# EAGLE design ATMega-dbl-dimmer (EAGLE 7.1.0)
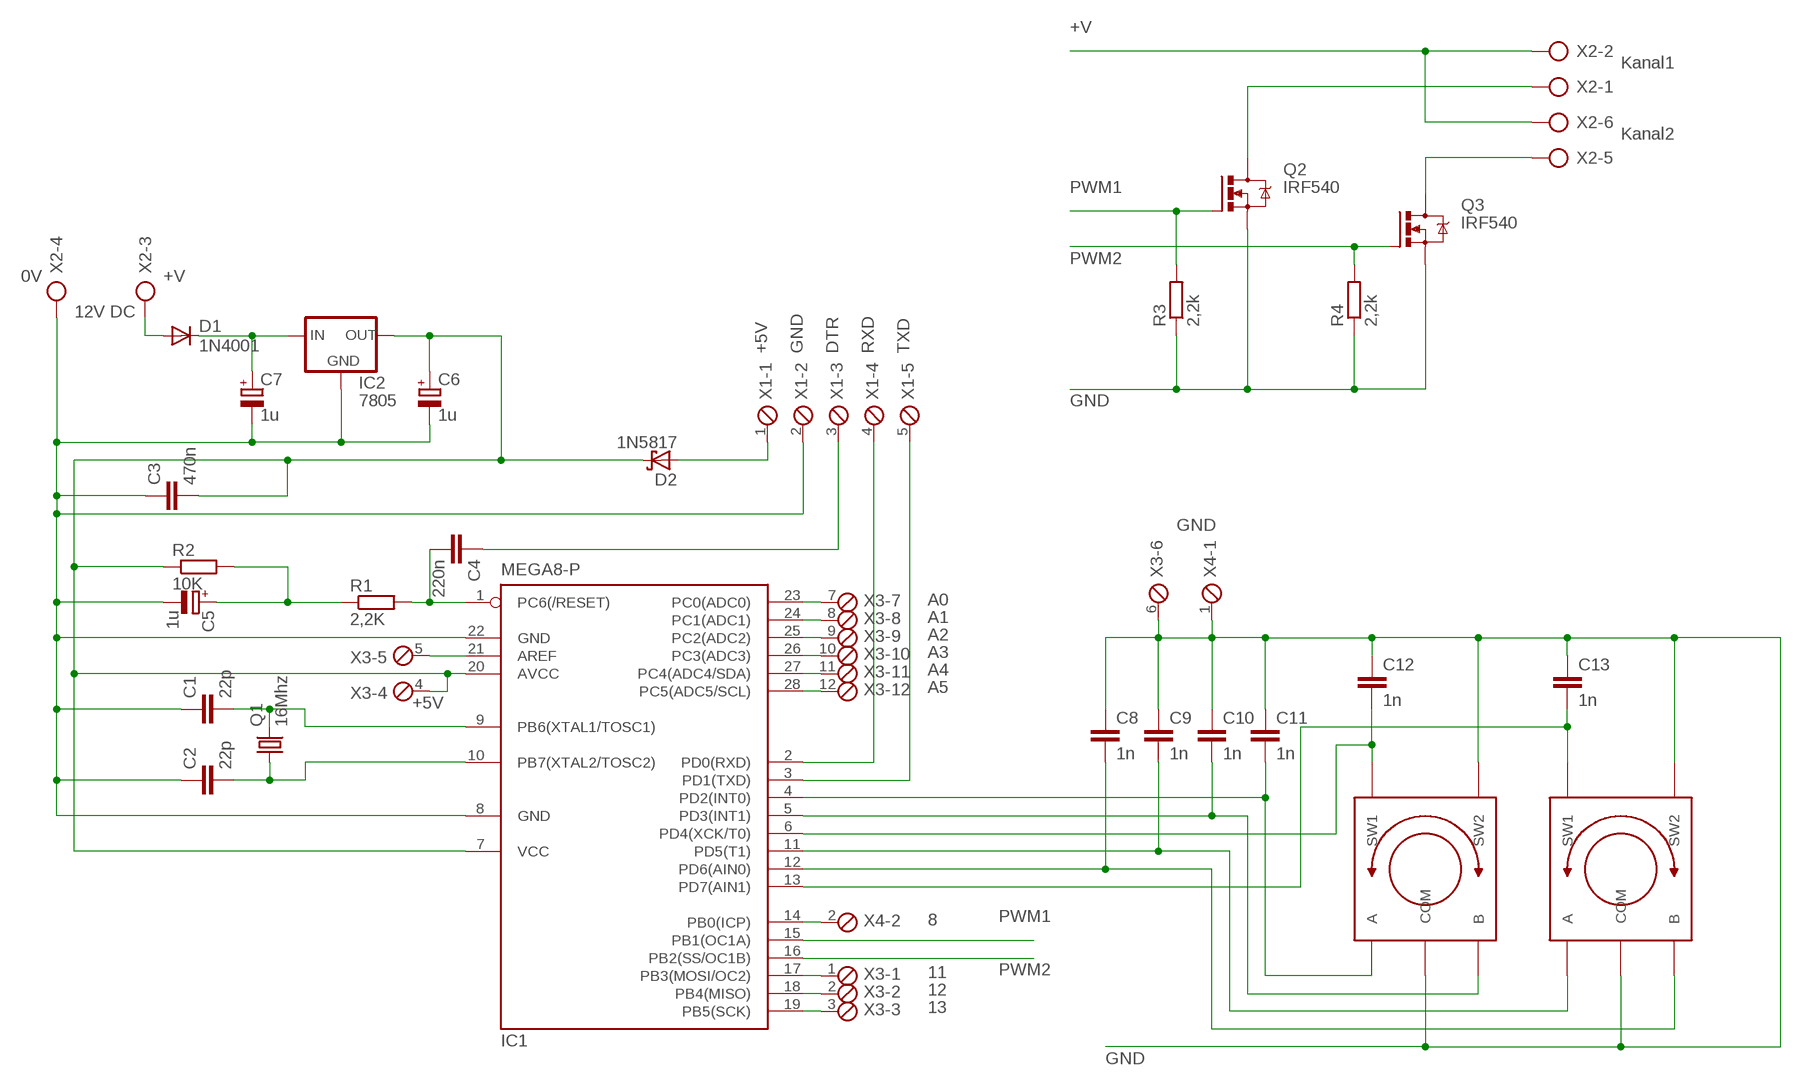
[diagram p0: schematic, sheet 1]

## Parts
C1  22p  C-EU025-025X050  [C025-025X050]
C2  22p  C-EU025-025X050  [C025-025X050]
C3  470n  C-EU075-042X103  [C075-042X103]
C4  220n  C-EU075-032X103  [C075-032X103]
C5  1u  CPOL-EUE5-6  [E5-6]
C6  1u  CPOL-EUE5-6  [E5-6]
C7  1u  CPOL-EUE5-6  [E5-6]
C8  1n  C-EU025-025X050  [C025-025X050]
C9  1n  C-EU025-025X050  [C025-025X050]
C10  1n  C-EU025-025X050  [C025-025X050]
C11  1n  C-EU025-025X050  [C025-025X050]
C12  1n  C-EU025-025X050  [C025-025X050]
C13  1n  C-EU025-025X050  [C025-025X050]
D1  1N4001  1N4004  [DO41-10]
D2  1N5817  1N5817-B  [DO41-7.6]
IC1  MEGA8-P  [DIL28-3]
IC2  7805  78XXS  [78XXS]
Q1  16Mhz  CRYSTALHC49S  [HC49/S]
Q2  IRF540  [TO220BV]
Q3  IRF540  [TO220BV]
R1  2,2K  R-EU_0207/7  [0207/7]
R2  10K  R-EU_0207/7  [0207/7]
R3  2,2k  R-EU_0207/7  [0207/7]
R4  2,2k  R-EU_0207/7  [0207/7]
S1  ROTARY-ENCODER  [RT-ENC-H]
S2  ROTARY-ENCODER  [RT-ENC-H]
X1  MPT5  [5POL254]
X2  AK300/6  [AK300/6]
X3  MPT12  [12POL254]
X4  MPT2  [2POL254]

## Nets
+5V: C3.2 C6.+ D2.C IC1.7(VCC) IC1.20(AVCC) IC2.OUT R2.1 X3.4
+V: D1.A X2.2 X2.3 X2.6
+V1: C7.+ D1.C IC2.IN
GND: C1.1 C2.1 C3.1 C5.- C6.- C7.- C8.1 C9.1 C10.1 C11.1 C12.1 C13.1 IC1.8(GND) IC1.22(GND) IC2.GND Q2.S Q3.S R3.1 R4.1 S1.P$2(COM) S1.P$5(SW2) S2.P$2(COM) S2.P$5(SW2) X1.2 X2.4 X3.6 X4.1
N$1: C1.2 IC1.9(PB6(XTAL1/TOSC1)) Q1.2
N$2: C2.2 IC1.10(PB7(XTAL2/TOSC2)) Q1.1
N$3: C4.2 IC1.1(PC6(/RESET)) R1.2
N$4: C5.+ R1.1 R2.2
N$7: IC1.2(PD0(RXD)) X1.4
N$8: IC1.3(PD1(TXD)) X1.5
N$9: C4.1 X1.3
N$10: C12.2 IC1.6(PD4(XCK/T0)) S1.P$4(SW1)
N$11: C13.2 IC1.13(PD7(AIN1)) S2.P$4(SW1)
N$12: C11.2 IC1.4(PD2(INT0)) S1.P$1(A)
N$13: C10.2 IC1.5(PD3(INT1)) S1.P$3(B)
N$14: C9.2 IC1.11(PD5(T1)) S2.P$1(A)
N$15: C8.2 IC1.12(PD6(AIN0)) S2.P$3(B)
N$16: Q3.D X2.5
N$17: Q2.D X2.1
N$19: IC1.21(AREF) X3.5
N$20: IC1.23(PC0(ADC0)) X3.7
N$21: IC1.24(PC1(ADC1)) X3.8
N$22: IC1.25(PC2(ADC2)) X3.9
N$23: IC1.26(PC3(ADC3)) X3.10
N$24: IC1.27(PC4(ADC4/SDA)) X3.11
N$25: IC1.28(PC5(ADC5/SCL)) X3.12
N$26: IC1.17(PB3(MOSI/OC2)) X3.1
N$27: IC1.18(PB4(MISO)) X3.2
N$28: IC1.19(PB5(SCK)) X3.3
N$29: IC1.14(PB0(ICP)) X4.2
N$30: D2.A X1.1
PWM1: IC1.15(PB1(OC1A)) Q2.G R3.2
PWM2: IC1.16(PB2(SS/OC1B)) Q3.G R4.2

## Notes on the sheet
- +V
- Kanal1
- Kanal2
- PWM1
- PWM2
- 0V | +V
- 12V DC
- +5V | GND | DTR | RXD | TXD
- GND
- GND
- A0
  A1
  A2
  A3
  A4
  A5
- +5V
- PWM1
- PWM2
- 8
  
  
  11
  12
  13
- GND

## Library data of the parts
C1-C4 C8-C13 = rcl:C-EU: CAPACITOR, European symbol
C5-C7 = rcl:CPOL-EU: POLARIZED CAPACITOR, European symbol
D1 = diode:1N4004: DIODE
D2 = diode:1N581*: 1.0A SCHOTTKY BARRIER RECTIFIER
IC1 = atmel:MEGA8-P: MICROCONTROLLER 8 Kbytes FLASH, 1 kbytes SRAM, 512 bytes EEPROM, USART, 4-channel 10 bit ADC, 2-channel 8 bit ADC Pin compatible with Atmega48, ATMega88, ATMega168 Source: avr.lbr; OC_FARNELL: unknown; OC_NEWARK: unknown
IC2 = v-reg:78XXS: VOLTAGE REGULATOR
Q1 = crystal:CRYSTAL: CRYSTAL; OC_FARNELL: 1667008; OC_NEWARK: unknown
Q2 Q3 = transistor-power:IRF540: HEXFET Power MOSFET
R1-R4 = rcl:R-EU_: RESISTOR, European symbol
S1 S2 = tormod:ROTARY-ENCODER
X1 = con-phoenix-254:MPT5: PHOENIX CONNECTOR; OC_FARNELL: unknown; OC_NEWARK: unknown
X2 = con-ptr500:AK300/6: CONNECTOR; OC_FARNELL: unknown; OC_NEWARK: unknown
X3 = con-phoenix-254:MPT12: PHOENIX CONNECTOR; OC_FARNELL: unknown; OC_NEWARK: unknown
X4 = con-phoenix-254:MPT2: PHOENIX CONNECTOR; OC_FARNELL: unknown; OC_NEWARK: unknown

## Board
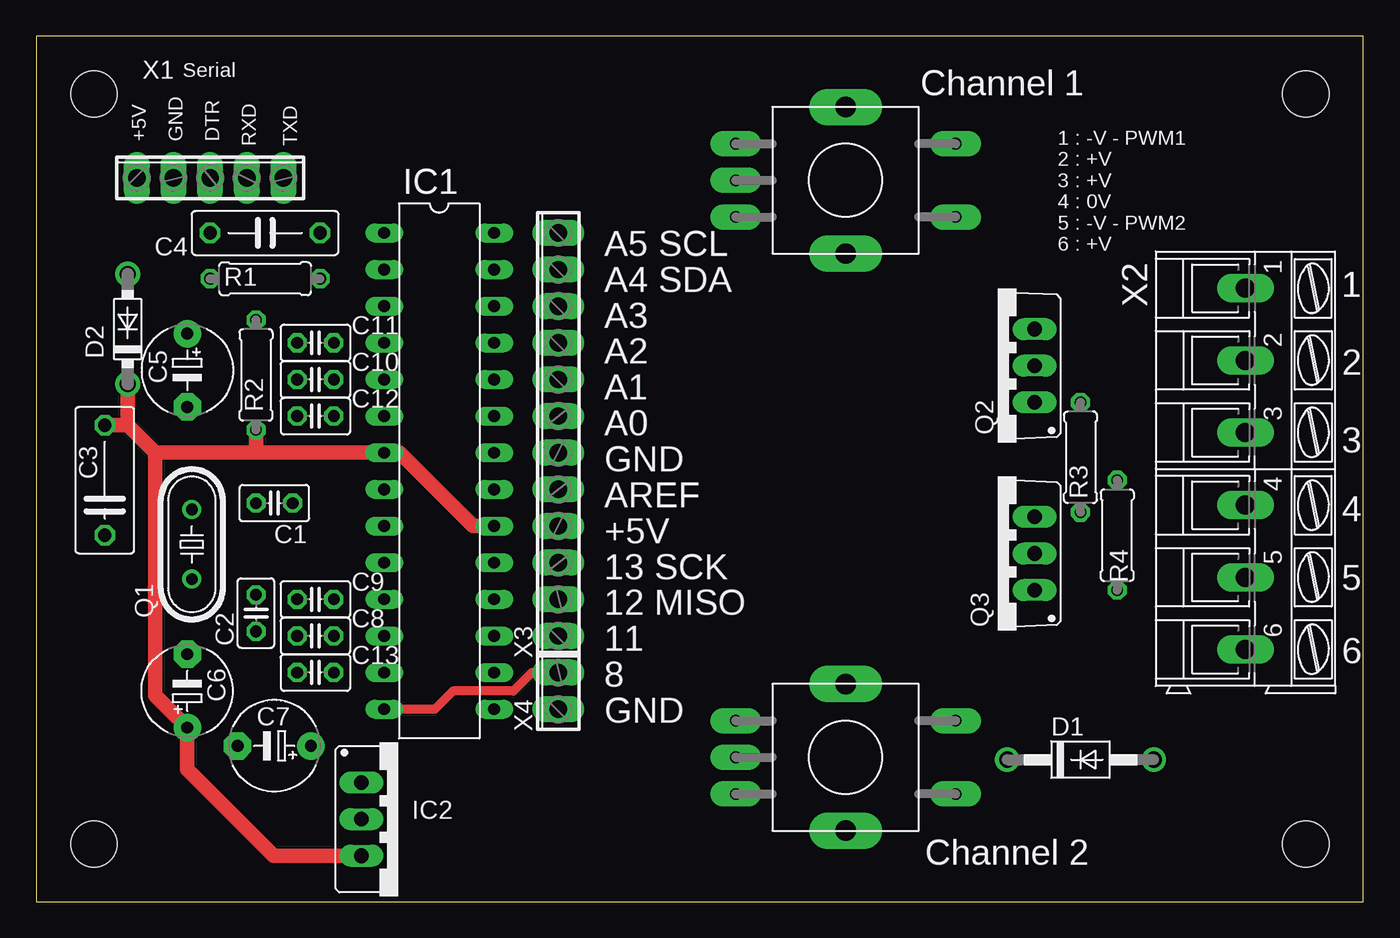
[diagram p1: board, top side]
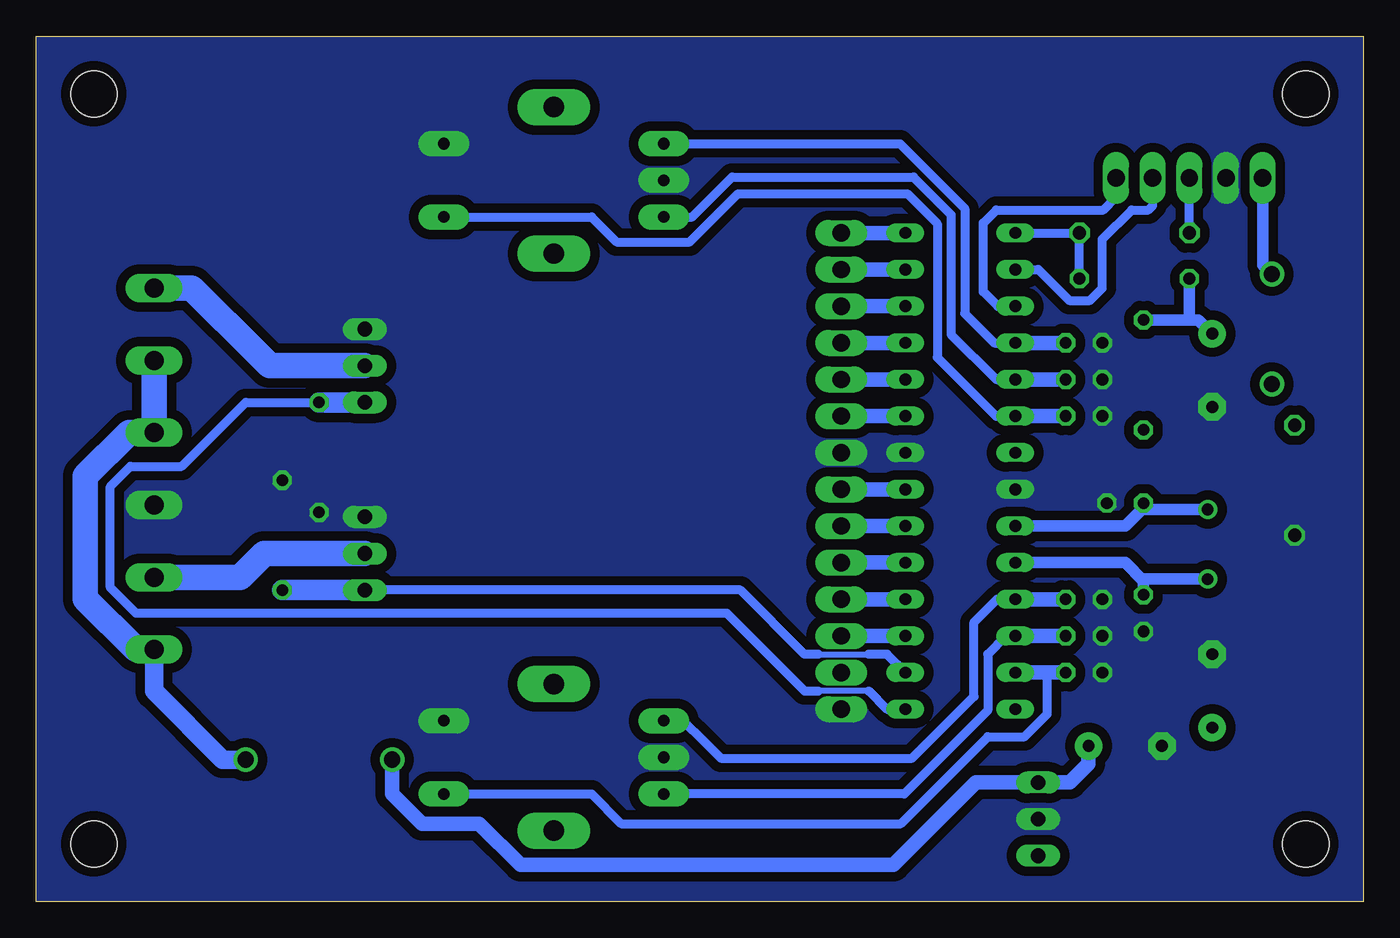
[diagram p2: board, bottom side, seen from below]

Size 92 x 60 mm. Coordinates in mm from the lower left corner, seen from the top.
Outline: 0,0 92,0 92,60 0,60 0,0
Copper layers (1*16): Top 0.035mm / dielectric 1.5mm / Bottom 0.035mm
Design rules "default *": minimum track width 10mil, minimum drill 24mil, track to track 8mil, track to pad 8mil, pad to pad 8mil, via to via 8mil, smd to smd 8mil, copper to edge 0mil, drill to drill 8mil, minimum pad ring 10mil, minimum via ring 8mil, stop-mask expansion 4mil, vias tented up to drill 0mil, thermal gap 10mil
Holes 3.2 mm at 4,56 88,56 88,4 4,4

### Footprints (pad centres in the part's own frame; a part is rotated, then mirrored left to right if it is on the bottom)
C025-025X050 = drill 0.813 octagon: 1 -1.27,0; 2 1.27,0
C075-042X103 = drill 0.914 octagon: 1 -3.81,0; 2 3.81,0
C075-032X103 = drill 0.914 octagon: 1 -3.81,0; 2 3.81,0
E5-6 = drill 0.813 pad 1.905: + -2.54,0 | drill 0.813 pad 1.905 octagon: - 2.54,0
DO41-10 = drill 1.118: A 5.08,0; C -5.08,0
DO41-7.6 = drill 1.1 pad 1.7: A 3.81,0; C -3.81,0
DIL28-3 = drill 0.813 long: 1 -16.51,-3.81; 2 -13.97,-3.81; 3 -11.43,-3.81; 4 -8.89,-3.81; 5 -6.35,-3.81; 6 -3.81,-3.81; 7 -1.27,-3.81; 8 1.27,-3.81; 9 3.81,-3.81; 10 6.35,-3.81; 11 8.89,-3.81; 12 11.43,-3.81; 13 13.97,-3.81; 14 16.51,-3.81; 15 16.51,3.81; 16 13.97,3.81; 17 11.43,3.81; 18 8.89,3.81; 19 6.35,3.81; 20 3.81,3.81; 21 1.27,3.81; 22 -1.27,3.81; 23 -3.81,3.81; 24 -6.35,3.81; 25 -8.89,3.81; 26 -11.43,3.81; 27 -13.97,3.81; 28 -16.51,3.81
78XXS = drill 1.016 long: GND 0,-2.54; IN -2.54,-2.54; OUT 2.54,-2.54
HC49/S = drill 0.813: 1 -2.413,0; 2 2.413,0
TO220BV = drill 1.016 long: D 0,-2.54; G -2.54,-2.54; S 2.54,-2.54
0207/7 = drill 0.813 octagon: 1 -3.81,0; 2 3.81,0
RT-ENC-H = drill 0.8 pad 1.778 long: P$1 -7.62,2.54; P$2 -7.62,0; P$3 -7.62,-2.54; P$4 7.62,-2.54; P$5 7.62,2.54 | drill 1.4 pad 2.54 long: P$6 0,5.08; P$7 0,-5.08
5POL254 = drill 1.2 long: 1 -5.08,0; 2 -2.54,0; 3 0,0; 4 2.54,0; 5 5.08,0
AK300/6 = drill 1.321 long: 1 -12.522,0; 2 -7.518,0; 3 -2.515,0; 4 2.515,0; 5 7.518,0; 6 12.522,0
12POL254 = drill 1.2 long: 1 -13.97,0; 2 -11.43,0; 3 -8.89,0; 4 -6.35,0; 5 -3.81,0; 6 -1.27,0; 7 1.27,0; 8 3.81,0; 9 6.35,0; 10 8.89,0; 11 11.43,0; 12 13.97,0
2POL254 = drill 1.2 long: 1 -1.27,0; 2 1.27,0

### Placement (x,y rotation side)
C1  16.51,27.62 180 top
C2  15.24,20 90 top
C3  4.76,29.21 90 top
C4  15.88,46.35 0 top
C5  10.48,36.83 270 top
C6  10.48,14.61 90 top
C7  16.51,10.79 180 top
C8  19.37,18.41 0 top
C9  19.37,20.95 0 top
C10  19.37,36.2 0 top
C11  19.37,38.73 0 top
C12  19.37,33.66 0 top
C13  19.37,15.88 0 top
D1  72.39,9.84 0 top
D2  6.35,39.69 90 top
IC1  27.94,29.84 270 top
IC2  25.08,5.71 270 top
Q1  10.79,24.77 90 top
Q2  66.67,37.15 90 top
Q3  66.67,24.13 90 top
R1  15.88,43.18 0 top
R2  15.24,36.51 90 top
R3  72.39,30.8 90 top
R4  74.93,25.4 270 top
S1  56.11,50 0 top
S2  56.11,10 0 top
X1  12.06,50.16 0 top
X2  83.82,30 270 top
X3  36.2,32.38 90 top
X4  36.2,14.61 90 top

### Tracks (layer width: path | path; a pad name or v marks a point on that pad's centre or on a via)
+5V
  Top 1.016: IC1.20 30.29,26.04 25.21,31.11 IC1.7 15.24,31.11 | 15.24,31.11 R2.1 | 15.24,31.11 8.26,31.11 | 8.26,31.11 6.35,33.02 | 6.35,33.02 D2.C | C3.2 6.35,33.02 | IC2.OUT 16.47,3.17 10.48,9.17 C6.+ 8.26,14.29 8.26,31.11
  Bottom 1.016: IC1.20 X3.4
+V
  Bottom 1.27: D1.A 79.06,9.84 83.82,14.61 X2.6
  Bottom 1.778: X2.6 85.08,17.48 88.58,20.98 88.58,29.49 85.56,32.52 X2.3 X2.2
+V1
  Bottom 1.016: D1.C 67.31,7.46 65.25,5.4 61.28,5.4 58.42,2.54 32.58,2.54 26.86,8.26 IC2.IN 20.36,8.26 19.05,9.56 C7.+
GND
  pour Bottom (isolate 0.65, no thermals): 0,0 92,0 92,60 0,60
N$1
  Bottom 0.813: IC1.9 16.51,26.04 15.4,27.15 15.37,27.18 | 15.37,27.18 Q1.2 | C1.2 15.24,27.3 15.37,27.18
N$2
  Bottom 0.813: IC1.10 16.51,23.5 15.24,22.23 | Q1.1 15.11,22.35 15.24,22.23 | C2.2 15.24,22.23
N$3
  Bottom 0.61: IC1.1 C4.2 R1.2
N$4
  Bottom 0.813: C5.+ 11.43,40.32 12.06,40.32 | 12.06,40.32 R2.2 | R1.1 12.06,40.32
N$7
  Bottom 0.61: IC1.2 22.54,43.81 20.39,41.67 18.94,41.67 18.1,42.51 18.1,45.91 16.07,47.94 14.92,47.94 14.61,48.26 X1.4
N$8
  Bottom 0.61: IC1.3 25.35,41.27 26.35,42.28 26.35,47.04 25.45,47.94 18.04,47.94 17.14,48.84 X1.5
N$9
  Bottom 0.61: C4.1 X1.3
N$10
  Bottom 0.61: IC1.6 25.46,33.66 29.53,37.72 29.53,46.99 31.61,49.08 43.34,49.08 46.7,45.72 51.75,45.72 53.49,47.46 S1.P$4
  Bottom 1.016: C12.2 IC1.6
N$11
  Bottom 0.61: S2.P$4 53.5,7.46 51.44,5.4 32.06,5.4 26.04,11.43 23.49,11.43 21.91,13.01 21.91,15.88
  Bottom 1.016: IC1.13 21.91,15.88 C13.2
N$12
  Bottom 0.61: S1.P$1 32.11,52.54 27.62,48.05 27.62,40.77 25.59,38.73 IC1.4
  Bottom 1.016: C11.2 IC1.4
N$13
  Bottom 0.61: S1.P$3 46.52,47.46 43.76,50.22 31.19,50.22 28.57,47.61 28.57,39.32 25.45,36.2 IC1.5
  Bottom 1.016: C10.2 IC1.5
N$14
  Bottom 0.61: S2.P$1 47.15,12.54 45.72,11.11 44.54,9.93 31.28,9.93 26.99,14.22 26.99,19.37 25.4,20.95 IC1.11
  Bottom 1.016: C9.2 IC1.11
N$15
  Bottom 0.61: S2.P$3 31.83,7.46 26.04,13.25 26.04,17.14 24.77,18.41 IC1.12
  Bottom 1.016: C8.2 IC1.12
N$16
  Bottom 1.778: Q3.D 76.2,24.13 77.85,22.48 X2.5
N$17
  Bottom 1.778: Q2.D 75.81,37.15 76.52,37.86 81.2,42.55 83.82,42.55 X2.1
N$19
  Bottom 1.016: X3.5 IC1.21
N$20
  Bottom 1.016: IC1.23 X3.7
N$21
  Bottom 1.016: IC1.24 X3.8
N$22
  Bottom 1.016: IC1.25 X3.9
N$23
  Bottom 1.016: X3.10 IC1.26
N$24
  Bottom 1.016: X3.11 IC1.27
N$25
  Bottom 1.016: X3.12 IC1.28
N$26
  Bottom 1.016: IC1.17 X3.1
N$27
  Bottom 1.016: IC1.18 X3.2
N$28
  Bottom 1.016: X3.3 IC1.19
N$29
  Top 0.61: X4.2 34.37,15.88 33.66,15.16 33.09,14.61 28.89,14.61 27.62,13.34 IC1.14
N$30
  Bottom 0.813: X1.1 6.99,44.13 D2.A
PWM1
  Bottom 0.406: 34.29,14.61 37.78,14.61
  Bottom 0.61: 34.29,14.61 33.02,13.34 IC1.15 | 37.78,14.61 38.73,14.61 44.13,20 85.09,20 86.86,21.77 86.86,28.77 85.46,30.16 81.92,30.16 77.47,34.61 R3.2
  Bottom 1.422: R3.2 Q2.G
PWM2
  Bottom 0.406: 37.78,17.14 34.29,17.14
  Bottom 0.61: IC1.16 33.02,17.14 34.29,17.14 | 37.78,17.14 38.73,17.14 43.18,21.59 Q3.G
  Bottom 1.422: R4.2 Q3.G

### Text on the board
tNames: Serial | Channel 1 | +5V | GND | DTR | RXD | TXD | 1 : -V - PWM1 / 2 : +V / 3 : +V / 4 : 0V / 5 : -V - PWM2 / 6 : +V | 1 | 2 | 3 | 4 | 5 | 6 | A5 SCL / A4 SDA / A3 / A2 / A1 / A0 / GND / AREF / +5V / 13 SCK / 12 MISO / 11 / 8 / GND | Channel 2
